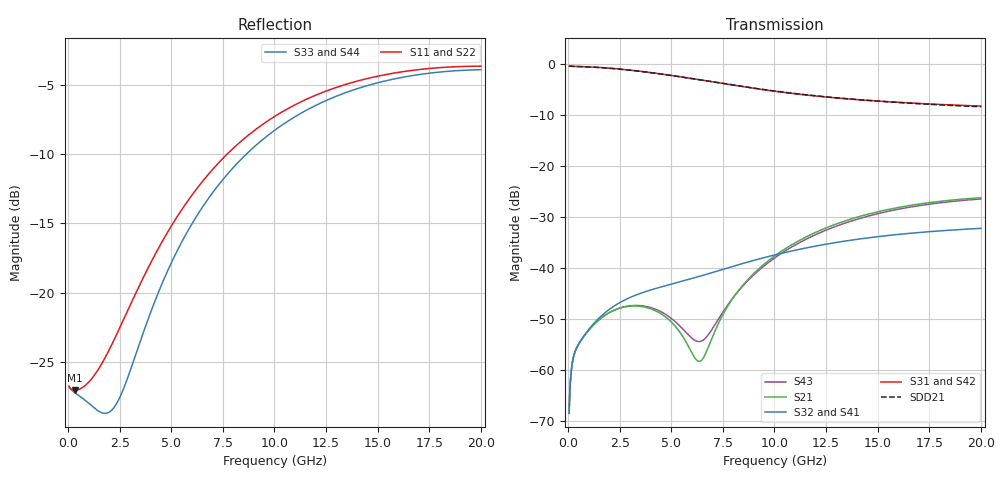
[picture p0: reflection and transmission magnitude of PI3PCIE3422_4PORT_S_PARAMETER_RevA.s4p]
! NPort=4 DATA=800 NOISE=0 GROUPDELAY=0 COMPLEX_DATAFORMAT=POLAR
! NumOfBlock=1 NumOfParam=0
! .MODEL Smodel S TSTONEFILE=PI3PCIE3422_4PORT_S_PARAMETER_RevA.s4p TYPE=S
!  -- The above .MODEL line can be used for the S element in the netlist.
! PORT DEFINITION
! PORT1 = INPUT+
! PORT2 = INPUT-
! PORT3 = OUTPUT+
! PORT4 = OUTPUT-
# Hz S MA R  50
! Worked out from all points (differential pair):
!   800 points, 50 MHz to 20 GHz, reference 50 ohm
!   strongest paths, dB at 50 MHz, 5.044 GHz, 10.04 GHz, 15.03 GHz, 20 GHz:
!     S31: -0.5, -2.3, -5.4, -7.3, -8.3
!     S42: -0.5, -2.3, -5.4, -7.3, -8.3
!     S32: -68.5, -43.2, -37.5, -33.9, -32.3
!     S41: -68.5, -43.2, -37.5, -33.9, -32.3
!     S21: -68.5, -50.8, -37.6, -29.0, -26.3
!     S43: -68.5, -50.1, -38.0, -29.4, -26.5
!   taken as a pair (ports 1,2 in; 3,4 out), SDD21 dB: -0.5, -2.3, -5.4, -7.3, -8.4
!   lowest |S11| = -27.1 dB at 349.6 MHz (marker M1), VSWR 1.09, Z = 54.2 - j1.86 ohm
!   |S11| at or under -10 dB: start of sweep to 7.715 GHz
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5e7  0.04587 -5.2  0.0003746 79.5  0.9463 -0.8  0.0003742 79.5
     0.0003746 79.5  0.04587 -5.2  0.0003742 79.5  0.9463 -0.8
     0.9463 -0.8  0.0003742 79.5  0.04587 -4.3  0.0003746 79.6
     0.0003742 79.5  0.9463 -0.8  0.0003746 79.6  0.04587 -4.3
3.49625e8  0.0444 -22.7  0.001528 49.4  0.9415 -4.7  0.001528 49.3
           0.001528 49.4  0.04441 -22.8  0.001528 49.3  0.9415 -4.7
           0.9415 -4.7  0.001528 49.3  0.04337 -16.5  0.001527 49.5
           0.001528 49.3  0.9415 -4.7  0.001527 49.5  0.04337 -16.5
3.04625e9  0.0913 -157.1  0.004209 36.4  0.8634 -38.3  0.005159 37.6
           0.00421 36.4  0.09156 -157.1  0.005159 37.6  0.8632 -38.3
           0.8634 -38.3  0.005159 37.6  0.05321 -163.3  0.00425 39.2
           0.00516 37.6  0.8633 -38.3  0.00425 39.2  0.05343 -163.3
5.76783e9  0.2125 130.1  0.001788 39.0  0.7272 -67.7  0.007605 23.8
           0.001788 39.0  0.2128 130.1  0.007605 23.7  0.727 -67.7
           0.7274 -67.7  0.007606 23.8  0.1652 119.3  0.002264 48.8
           0.007607 23.8  0.7271 -67.7  0.002264 48.8  0.1654 119.4
6.46696e9  0.2493 116.2  0.00124 94.0  0.6908 -74.4  0.008346 20.8
           0.001239 94.0  0.2497 116.2  0.008346 20.8  0.6905 -74.4
           0.6909 -74.3  0.008347 20.9  0.201 106.5  0.001914 85.7
           0.008348 20.9  0.6906 -74.4  0.001913 85.7  0.2013 106.5
1.15855e10  0.4995 39.3  0.02031 123.6  0.492 -113.6  0.01571 -15.7
            0.02031 123.6  0.4998 39.3  0.01571 -15.7  0.4918 -113.6
            0.4922 -113.6  0.01572 -15.7  0.4563 35.8  0.01929 119.9
            0.01572 -15.7  0.492 -113.5  0.01929 119.9  0.4566 35.8
2e10  0.6556 -32.1  0.04854 67.9  0.3844 -173.1  0.02431 -99.1
      0.04854 67.9  0.6558 -32.1  0.02431 -99.1  0.3843 -173.1
      0.3847 -173.0  0.02433 -99.0  0.6365 -32.9  0.04722 67.8
      0.02433 -99.0  0.3846 -173.0  0.04722 67.8  0.6366 -32.9
